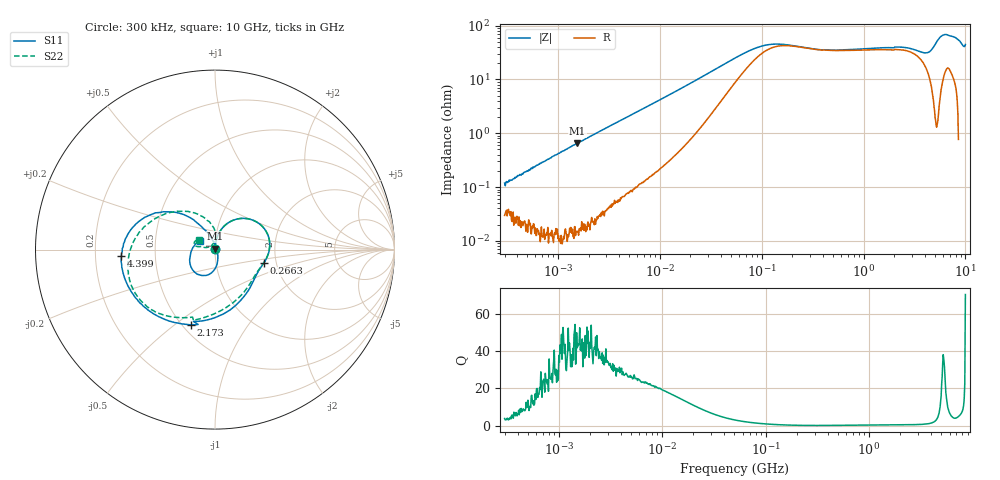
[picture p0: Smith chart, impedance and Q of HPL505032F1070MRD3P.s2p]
! S-Parameter Data Generated by TDK Corporation
! Copyright(C) 2024 TDK Corporation.
! All Rights Reserved.
! TDK P/N: HPL505032F1070MRD3P (SMD / SMT Inductor (Coil))
! Property: L=70nH at 100kHz
! Size(LxWxT): 5x5x3.2mm
! Model Type: s2p (Touchstone File Format Version 1.0)
! Frequency: DC=Yes Start=0.3MHz Stop=10000MHz 802points Log-sweep
! Model Generated on May 28, 2024
! Terms and conditions regarding TDK Simulation Models:
! 1)This simulation model is being provided solely for informational
!  purposes. Please refer to the specifications of the products in
!  terms of detailed characteristics of such products.
! 2)In no event shall TDK Corporation of any of its subsidiaries be
!  liable for any loss or damage arising, directly or indirectly,
!  from any information contained in this simulation model, including,
!  but not limited to loss or damages arising from any inaccuracies,
!  omissions or errors in connection with such information.
! 3)Any and all copyrights on this simulation model are owned by
!  TDK Corporation.  Duplication or redistribution of this simulation
!  model without prior written permission from TDK Corporation
!  is prohibited.
! 4)This simulation model is subject to any modification or change
!  without any prior notice.
! 5)Neither TDK Corporation nor any of its subsidiaries shall make any
!  warranty, express or implied, including but not limited to the
!  correctness, implied warranties of merchantability and fitness for
!  a particular purpose with respect to this simulation models.
! 6)The use of this simulation model shall be deemed to have consented
!  to the terms and conditions hereof.
! Port Assignments:
!  1 ---@@@--- 2
! Applicable Conditions:
!  Temperature = 25 degC
!  DC Bias Current = 0 A
!  Small Signal Operation
# Hz S MA R 50
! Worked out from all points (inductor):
!   801 points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, 300 kHz to 10 GHz, reference 50 ohm
!   read as one part in series: L = 62 nH near 318.3 kHz
!   highest Q = 44.6 at 1.55 MHz (marker M1), where L = 66.5 nH
!   S11 on the Smith chart (normalised r, x): 300 kHz: 1.00, +0.00; 266.3 MHz: 1.71, -0.28; 2.173 GHz: 0.55, -0.57; 4.399 GHz: 0.31, -0.03; 10 GHz: 0.84, +0.08
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300000  0.001073 70.5  0.9997 -0.1  0.9996 -0.0  0.001218 79.7
1550270  0.005926 88.1  0.9998 -0.4  0.9999 -0.4  0.005956 88.5
1713600  0.006574 87.7  0.9998 -0.4  0.9996 -0.4  0.006668 88.3
9671944  0.03674 84.4  0.9972 -2.5  0.9974 -2.5  0.03677 84.4
5.477226e7  0.209 54.4  0.9023 -13.4  0.9024 -13.4  0.2088 54.5
1.063884e8  0.3006 21.3  0.7407 -14.5  0.7408 -14.5  0.3003 21.4
2.663116e8  0.2814 -15.8  0.7175 -8.9  0.7177 -8.9  0.2805 -15.7
3.126428e8  0.2749 -20.3  0.725 -9.8  0.7252 -9.8  0.2733 -20.2
8.299813e8  0.2967 -52.4  0.7047 -25.2  0.7048 -25.2  0.2835 -53.5
1.767019e9  0.3962 -97.2  0.5783 -50.4  0.5782 -50.4  0.3823 -98.9
2.172958e9  0.4395 -107.8  0.5145 -58.7  0.5145 -58.7  0.411 -112.8
3.135132e9  0.5026 -137.9  0.3764 -73.9  0.3763 -73.9  0.4884 -137.0
4.399376e9  0.523 -175.9  0.2267 -78.9  0.2271 -78.8  0.4945 -168.7
5.21579e9  0.4632 162.1  0.1855 -61.9  0.1862 -61.9  0.434 167.2
6.091595e9  0.3023 136.6  0.2536 -46.0  0.2542 -46.2  0.3121 137.7
6.737565e9  0.1481 120.3  0.3518 -49.6  0.352 -49.8  0.2081 113.8
7.141296e9  0.06732 106.9  0.4254 -57.7  0.4251 -57.8  0.1442 98.9
7.316673e9  0.02972 92.7  0.4535 -62.4  0.4542 -62.6  0.1215 93.1
7.763894e9  0.06156 -75.6  0.5099 -75.3  0.5101 -75.5  0.06046 89.9
8.09931e9  0.1168 -93.3  0.538 -85.9  0.5384 -86.1  0.02979 129.4
8.881947e9  0.1694 -126.1  0.5397 -109.6  0.5396 -109.7  0.08969 169.9
1e10  0.09582 149.0  0.4382 -143.7  0.4381 -143.9  0.1039 149.3
